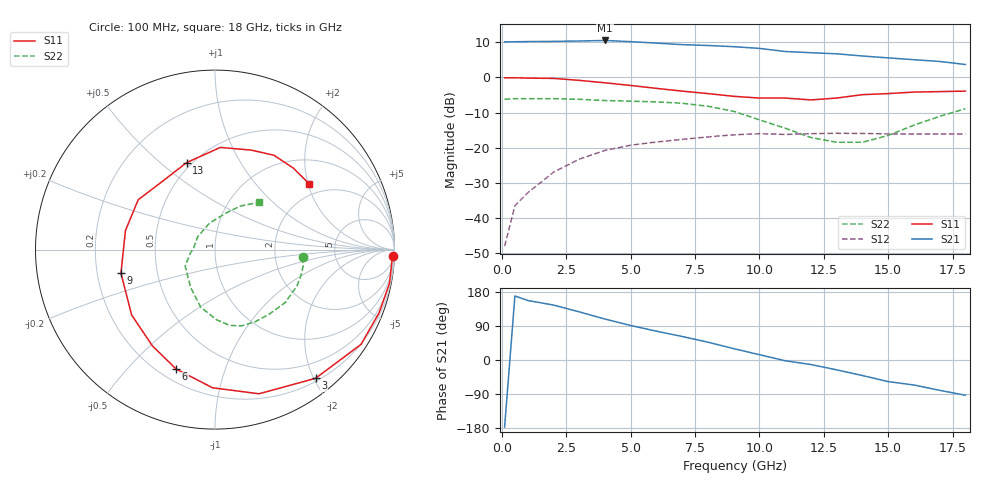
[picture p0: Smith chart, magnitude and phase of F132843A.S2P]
!ATF-13284
!S-PARAMETERS at Vds=2.5V  Id=20mA.  LAST UPDATED 07-22-92
# ghz s ma r 50
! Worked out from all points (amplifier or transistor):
!   20 points, 100 MHz to 18 GHz, reference 50 ohm
!   highest |S21| = 10.5 dB at 4 GHz (marker M1)
!   |S21| within 3 dB of that: start of sweep to 10.84 GHz
!   unconditionally stable (mu >= 1): 10.36 GHz to end of sweep
!   at 2 GHz: K = 0.23, MSG = 18.6 dB, |S12| = -26.9 dB
!   at 9 GHz: K = 0.89, MSG = 12.5 dB, |S12| = -16.3 dB
!   at 18 GHz: K = 1.23, MAG = 7.0 dB, |S12| = -16.1 dB
!   lowest NFmin = 0.60 dB at 500 MHz
!   S11 on the Smith chart (normalised r, x): 100 MHz: 15, -53; 3 GHz: 0.24, -2.03; 6 GHz: 0.27, -0.69; 9 GHz: 0.30, -0.11; 13 GHz: 0.47, +0.62; 18 GHz: 1.64, +2.03
0.1  0.99 -2.0  3.21 -177.0  0.004 95.0  0.49 -5.0
0.5  0.99 -11.0  3.22 169.0  0.015 80.0  0.5 -11.0
1  0.98 -21.0  3.24 157.0  0.023 74.0  0.5 -17.0
2  0.97 -33.0  3.26 145.0  0.045 67.0  0.5 -24.0
3  0.91 -52.0  3.3 127.0  0.069 55.0  0.49 -37.0
4  0.84 -73.0  3.36 108.0  0.092 42.0  0.47 -50.0
5  0.77 -91.0  3.23 91.0  0.109 31.0  0.46 -61.0
6  0.7 -108.0  3.08 76.0  0.121 22.0  0.45 -71.0
7  0.64 -123.0  2.93 62.0  0.132 14.0  0.43 -79.0
8  0.59 -142.0  2.85 47.0  0.143 5.0  0.39 -89.0
9  0.54 -166.0  2.74 30.0  0.153 -5.0  0.33 -104.0
10  0.51 168.0  2.59 14.0  0.159 -15.0  0.25 -123.0
11  0.51 147.0  2.34 -2.0  0.155 -22.0  0.19 -151.0
12  0.48 127.0  2.25 -12.0  0.159 -30.0  0.14 -171.0
13  0.51 108.0  2.17 -26.0  0.161 -35.0  0.12 177.0
14  0.57 87.0  2.02 -41.0  0.16 -46.0  0.12 144.0
15  0.59 70.0  1.9 -57.0  0.158 -53.0  0.15 102.0
16  0.62 58.0  1.79 -66.0  0.157 -59.0  0.21 74.0
17  0.63 46.0  1.69 -80.0  0.157 -67.0  0.28 60.0
18  0.64 35.0  1.53 -93.0  0.157 -84.0  0.36 47.0
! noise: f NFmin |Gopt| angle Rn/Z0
0.5  0.6  0.96  5  1.4
1  0.6  0.92  10  1.3
2  0.6  0.85  21  1.2
4  0.7  0.75  54  1
6  1  0.66  99  0.7
8  1.2  0.57  144  0.3
12  1.6  0.51  -116  0.1
15  2.4  0.55  -52  0.5
